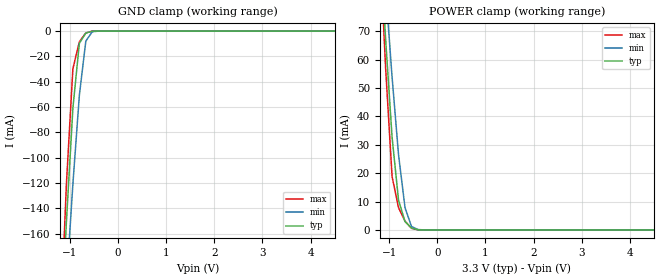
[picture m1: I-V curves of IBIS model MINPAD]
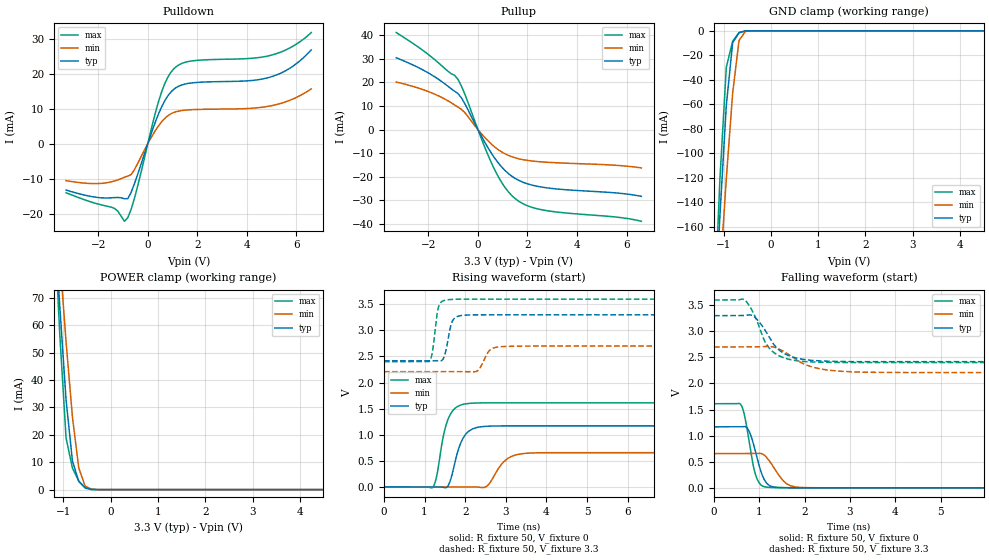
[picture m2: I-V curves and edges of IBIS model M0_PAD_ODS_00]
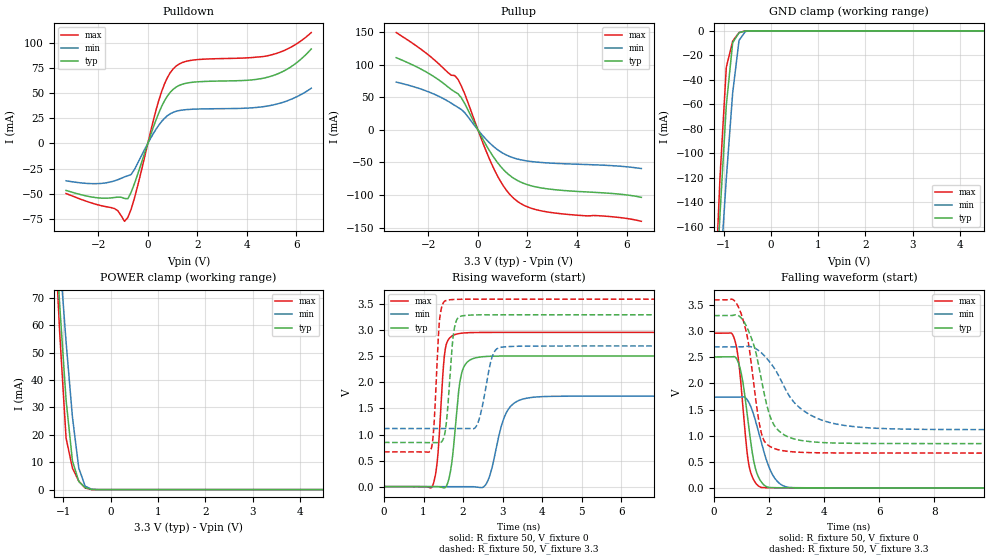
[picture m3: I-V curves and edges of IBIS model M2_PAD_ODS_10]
| Created by SiliconSmart  O-2018.09-SP2-3
[IBIS Ver]   4.0
[File Name]   as31b32bc_3p3_rev1p4.ibs
[File Rev]   1.4
[Date]   Thursday Mar 21 2024
|[Source]   Avalanche Team
|[Notes]   Generated IBIS models from Silicon Smart
|[Rev 1.0]  Initial Release based on extracted netlist
|   Characterization
|[Rev 1.1]  Recharacterization with Hspice, run in high accuracy mode
|[Rev 1.2]  Recharacterization with Hspice, run with parameters inline
|   with the datasheet
|[Rev 1.3]  Recharacterization with Hspice, run with updated VIH/VIL
|   in parallel with datasheet rev X.7
|[Rev 1.4]  Update the pin to the package pinout assignment
|[Disclaimer]   THE MODEL LIBRARIES ARE PROVIDED AS IS.
|[Copyright]   Copyright 2019, Avalanche Technology., All Rights Reserved
[Component]   AS301GB32_BGA
[Manufacturer] Avalanche Technology
| CONTENT :
| This file contains IBIS MODEL for PSRAM device
| AS301GB32
| USAGE :
| The models are derived for the 2.7V to 3.6V I/O Operation.
| Temperatures for model generation: typ: 25, max: -40, min: 125
| Voltages : typ: 3.3V, min: 2.7V, max: 3.6V
| PACKAGES SUPPORTED :
| 142-ball FBGA (15mm x 17mm)
| VERIFICATION
| Errors  : 0
| Warnings: 11
| All warnings due to non-monotonic data:
[Package]
R_pkg  0   0   0
L_pkg  0   0   0
C_pkg  0   0   0
[Pin]   signal_name   model_name   R_pin   L_pin   C_pin
P8   E#   MINPAD   0.254	7.307E-9	1.178E-12
P7   G#   MINPAD   0.243	7.052E-9	1.094E-12
J2   CR#   MINPAD   0.547	10.386E-9	1.789E-12
K3   PG#   MINPAD   0.451	10.329E-9	1.676E-12
M8   W#   MINPAD   0.377	9.020E-9	1.417E-12
M2   ADDR_26   MINPAD   0.425	9.037E-9	1.604E-12
L4   ADDR_25   MINPAD   0.419	9.644E-9	1.527E-12
K13   ADDR_24   MINPAD   0.495	9.978E-9	1.745E-12
M3   ADDR_23   MINPAD   0.371	9.313E-9	1.466E-12
L3   ADDR_22   MINPAD   0.412	9.753E-9	1.540E-12
M7   ADDR_21   MINPAD   0.368	8.765E-9	1.384E-12
P12   ADDR_20   MINPAD   0.287	8.287E-9	1.639E-12
L12   ADDR_19   MINPAD   0.424	10.320E-9	1.620E-12
N11   ADDR_18   MINPAD   0.338	8.691E-9	1.470E-12
N6   ADDR_17   MINPAD   0.309	8.196E-9	1.279E-12
P6   ADDR_16   MINPAD   0.256	7.462E-9	1.204E-12
L13   ADDR_15   MINPAD   0.463	10.719E-9	1.740E-12
M13   ADDR_14   MINPAD   0.421	10.290E-9	1.689E-12
P10   ADDR_13   MINPAD   0.262	7.671E-9	1.349E-12
N10   ADDR_12   MINPAD   0.340	8.540E-9	1.360E-12
M12   ADDR_11   MINPAD   0.402	9.876E-9	1.604E-12
N13   ADDR_10   MINPAD   0.399	9.819E-9	1.696E-12
L11   ADDR_9   MINPAD   0.443	9.732E-9	1.569E-12
M11   ADDR_8   MINPAD   0.436	9.682E-9	1.671E-12
P5   ADDR_7   MINPAD   0.253	7.464E-9	1.277E-12
P3   ADDR_6   MINPAD   0.279	8.031E-9	1.557E-12
N5   ADDR_5   MINPAD   0.313	8.320E-9	1.359E-12
N4   ADDR_4   MINPAD   0.329	8.138E-9	1.428E-12
M4   ADDR_3   MINPAD   0.379	8.543E-9	1.406E-12
N2   ADDR_2   MINPAD   0.378	9.572E-9	1.637E-12
N9   ADDR_1   MINPAD   0.315	8.416E-9	1.305E-12
M9   ADDR_0   MINPAD   0.403	9.225E-9	1.473E-12
E2   DQ_31   MIOPAD   0.365	8.798E-9	1.454E-12
F2   DQ_30   MIOPAD   0.418	9.057E-9	1.576E-12
D2   DQ_29   MIOPAD   0.358	8.697E-9	1.520E-12
E3   DQ_28   MIOPAD   0.348	8.812E-9	1.441E-12
E12   DQ_27   MIOPAD   0.327	8.506E-9	1.443E-12
D10   DQ_26   MIOPAD   0.309	7.715E-9	1.264E-12
C9   DQ_25   MIOPAD   0.279	7.395E-9	1.219E-12
C7   DQ_24   MIOPAD   0.252	6.802E-9	1.108E-12
G4   DQ_23   MIOPAD   0.455	10.071E-9	1.775E-12
G3   DQ_22   MIOPAD   0.457	10.100E-9	1.750E-12
F13   DQ_21   MIOPAD   0.377	9.387E-9	1.566E-12
D13   DQ_20   MIOPAD   0.295	8.231E-9	1.460E-12
C10   DQ_19   MIOPAD   0.293	7.553E-9	1.298E-12
E8   DQ_18   MIOPAD   0.393	8.323E-9	1.436E-12
F6   DQ_17   MIOPAD   0.425	8.913E-9	1.517E-12
E5   DQ_16   MIOPAD   0.379	8.982E-9	1.460E-12
E13   DQ_15   MIOPAD   0.363	8.555E-9	1.474E-12
G11   DQ_14   MIOPAD   0.475	9.536E-9	1.630E-12
E10   DQ_13   MIOPAD   0.404	8.563E-9	1.453E-12
F9   DQ_12   MIOPAD   0.409	9.347E-9	1.513E-12
C8   DQ_11   MIOPAD   0.257	6.782E-9	1.111E-12
C6   DQ_10   MIOPAD   0.238	7.000E-9	1.114E-12
D6   DQ_9   MIOPAD   0.292	7.776E-9	1.248E-12
D4   DQ_8   MIOPAD   0.305	7.782E-9	1.343E-12
G12   DQ_7   MIOPAD   0.502	10.055E-9	1.687E-12
C12   DQ_6   MIOPAD   0.275	7.857E-9	1.346E-12
D11   DQ_5   MIOPAD   0.286	7.835E-9	1.360E-12
D9   DQ_4   MIOPAD   0.306	8.035E-9	1.299E-12
E7   DQ_3   MIOPAD   0.384	8.178E-9	1.375E-12
C5   DQ_2   MIOPAD   0.231	6.786E-9	1.150E-12
D5   DQ_1   MIOPAD   0.307	7.698E-9	1.346E-12
C3   DQ_0   MIOPAD   0.267	7.420E-9	1.241E-12
G13   INT#   MIOPAD   0.480	10.704E-9	1.759E-12
F10   VSSIO   GND   NA   NA   NA
L10   VSSIO   GND   NA   NA   NA
E9   VSSIO   GND   NA   NA   NA
L9   VSSIO   GND   NA   NA   NA
F8   VSSIO   GND   NA   NA   NA
L8   VSSIO   GND   NA   NA   NA
F7   VSSIO   GND   NA   NA   NA
L7   VSSIO   GND   NA   NA   NA
E6   VSSIO   GND   NA   NA   NA
L6   VSSIO   GND   NA   NA   NA
G5   VSSIO   GND   NA   NA   NA
A14   VSS   GND   NA   NA   NA
B14   VSS   GND   NA   NA   NA
C14   VSS   GND   NA   NA   NA
H13   VSS   GND   NA   NA   NA
R14   VSS   GND   NA   NA   NA
T14   VSS   GND   NA   NA   NA
A13   VSS   GND   NA   NA   NA
T13   VSS   GND   NA   NA   NA
A12   VSS   GND   NA   NA   NA
G10   VSS   GND   NA   NA   NA
H10   VSS   GND   NA   NA   NA
J10   VSS   GND   NA   NA   NA
K10   VSS   GND   NA   NA   NA
F5   VSS   GND   NA   NA   NA
L5   VSS   GND   NA   NA   NA
A2   VSS   GND   NA   NA   NA
T2   VSS   GND   NA   NA   NA
A1   VSS   GND   NA   NA   NA
B1   VSS   GND   NA   NA   NA
R1   VSS   GND   NA   NA   NA
T1   VSS   GND   NA   NA   NA
F12   VCCIO   POWER   NA   NA   NA
J12   VCCIO   POWER   NA   NA   NA
E11   VCCIO   POWER   NA   NA   NA
M10   VCCIO   POWER   NA   NA   NA
D8   VCCIO   POWER   NA   NA   NA
N8   VCCIO   POWER   NA   NA   NA
D7   VCCIO   POWER   NA   NA   NA
N7   VCCIO   POWER   NA   NA   NA
M5   VCCIO   POWER   NA   NA   NA
E4   VCCIO   POWER   NA   NA   NA
F3   VCCIO   POWER   NA   NA   NA
J3   VCCIO   POWER   NA   NA   NA
C13   VCC   POWER   NA   NA   NA
P13   VCC   POWER   NA   NA   NA
D12   VCC   POWER   NA   NA   NA
N12   VCC   POWER   NA   NA   NA
C11   VCC   POWER   NA   NA   NA
F11   VCC   POWER   NA   NA   NA
H11   VCC   POWER   NA   NA   NA
J11   VCC   POWER   NA   NA   NA
K11   VCC   POWER   NA   NA   NA
P11   VCC   POWER   NA   NA   NA
C4   VCC   POWER   NA   NA   NA
F4   VCC   POWER   NA   NA   NA
H4   VCC   POWER   NA   NA   NA
J4   VCC   POWER   NA   NA   NA
K4   VCC   POWER   NA   NA   NA
P4   VCC   POWER   NA   NA   NA
D3   VCC   POWER   NA   NA   NA
N3   VCC   POWER   NA   NA   NA
C2   VCC   POWER   NA   NA   NA
P2   VCC   POWER   NA   NA   NA
| IOPAD
[Model Selector] MIOPAD
| Model Description
M0_PAD_ODS_00   ODS_00
M1_PAD_ODS_01   ODS_01
M2_PAD_ODS_10   ODS_10
M3_PAD_ODS_11   ODS_11
| Models and submodels in the file (5): MINPAD (Input), M0_PAD_ODS_00 (I/O), M2_PAD_ODS_10 (I/O), M1_PAD_ODS_01 (I/O), M3_PAD_ODS_11 (I/O)
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[Model] MINPAD
Model_type Input
Enable   Active-High
Vinl  =  0.8
Vinh  =  2.2
| Capacitance  typ   min   max
C_comp   1.514821e-12   1.418868e-12   1.647023e-12
| Variables   typ   min   max
[GND Clamp Reference]   0   0   0
[POWER Clamp Reference]   3.3   2.7   3.6
[Pulldown Reference]   0   0   0
[Pullup Reference]   3.3   2.7   3.6
[Temperature Range]   25   125   -40
[Voltage Range]   3.3   2.7   3.6
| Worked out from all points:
|   GND clamp passes 1 mA (typ) near -0.62 V on its own axis
|   POWER clamp passes 1 mA (typ) near -0.56 V on its own axis
[GND Clamp]
| Voltage   I(typ)   I(min)   I(max)
-3.3V     -1.961A    -1.697A    -2.357A
-1.21V    -250.7mA   -283.7mA   -242.5mA
-1.076V   -150.6mA   -200.1mA   -120.6mA
-941.4mV  -60.83mA   -120.8mA   -29.75mA
-806.9mV  -9.646mA   -50.71mA   -8.435mA
-672.4mV  -1.585mA   -7.866mA   -1.457mA
-537.9mV  -71.75uA   -504.3uA   -18.73uA
-403.4mV  -593.9nA   -18.57uA   -37.22nA
6.6V      0A         0A         0A
[POWER Clamp]
| Voltage   I(typ)   I(min)   I(max)
-3.3V     772.3mA    673.3mA    930.5mA
-1.21V    105.9mA    117.6mA    104.6mA
-1.076V   67.34mA    85.06mA    57.16mA
-941.4mV  32.71mA    53.93mA    18.82mA
-806.9mV  10.48mA    26.53mA    7.848mA
-672.4mV  2.975mA    7.856mA    3.108mA
-537.9mV  710.9uA    1.248mA    573.1uA
-403.4mV  60.69uA    160.8uA    9.187uA
-269mV    142.4nA    6.118uA    23.26nA
6.6V      0A         0A         0A
[Model] M0_PAD_ODS_00
Model_type I/O
Enable   Active-High
Vinl  =  0.8
Vinh  =  2.2
Vmeas =  1.65
Cref  =  30e-12
| Capacitance  typ   min   max
C_comp   1.518749e-12   1.424706e-12   1.652746e-12
| Variables   typ   min   max
[GND Clamp Reference]   0   0   0
[POWER Clamp Reference]   3.3   2.7   3.6
[Pulldown Reference]   0   0   0
[Pullup Reference]   3.3   2.7   3.6
[Temperature Range]   25   125   -40
[Voltage Range]   3.3   2.7   3.6
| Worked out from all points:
|   slope of the pulldown table from 0 to 0.495 V, typ, clamps not added: 52.1 ohm
|   slope of the pullup table from 0 to 0.495 V, typ, clamps not added: 53.8 ohm
|   GND clamp passes 1 mA (typ) near -0.62 V on its own axis
|   POWER clamp passes 1 mA (typ) near -0.56 V on its own axis
|   falling waveform, R_fixture 50, V_fixture 0: 20-80 % time 230ps typ, 320ps min, 198ps max; typ from 1.17 V to 0 V
|   falling waveform, R_fixture 50, V_fixture 3.3: 20-80 % time 464ps typ, 644ps min, 396ps max; typ from 3.3 V to 2.42 V
|   rising waveform, R_fixture 50, V_fixture 0: 20-80 % time 273ps typ, 362ps min, 248ps max; typ from 0 V to 1.17 V
|   rising waveform, R_fixture 50, V_fixture 3.3: 20-80 % time 138ps typ, 198ps min, 114ps max; typ from 2.42 V to 3.3 V
[GND Clamp]
| Voltage   I(typ)   I(min)   I(max)
-3.3V     -1.961A    -1.697A    -2.357A
-1.21V    -250.7mA   -283.7mA   -242.5mA
-1.076V   -150.6mA   -200.1mA   -120.7mA
-941.4mV  -60.83mA   -120.8mA   -29.76mA
-806.9mV  -9.649mA   -50.71mA   -8.442mA
-672.4mV  -1.587mA   -7.866mA   -1.46mA
-537.9mV  -71.93uA   -504.3uA   -18.83uA
-403.4mV  -595.6nA   -18.58uA   -37.45nA
6.6V      0A         0A         0A
[POWER Clamp]
| Voltage   I(typ)   I(min)   I(max)
-3.3V     772.3mA    673.3mA    930.5mA
-1.21V    105.9mA    117.6mA    104.6mA
-1.076V   67.34mA    85.06mA    57.16mA
-941.4mV  32.71mA    53.93mA    18.82mA
-806.9mV  10.48mA    26.53mA    7.848mA
-672.4mV  2.975mA    7.856mA    3.108mA
-537.9mV  710.9uA    1.248mA    573.1uA
-403.4mV  60.69uA    160.8uA    9.187uA
-269mV    142.4nA    6.118uA    23.26nA
6.6V      0A         0A         0A
[Pulldown]
| Voltage   I(typ)   I(min)   I(max)
-3.3V     -13.26mA   -10.58mA   -14.05mA
-1.345V   -15.42mA   -10.67mA   -18.51mA
-941.4mV  -15.74mA   -9.611mA   -22.19mA
-806.9mV  -15.73mA   -9.263mA   -21.14mA
-537.9mV  -11.42mA   -7.417mA   -15.59mA
455.2mV   8.881mA    5.308mA    12.55mA
682.8mV   12.23mA    7.205mA    17.1mA
1.024V    15.38mA    8.837mA    21.2mA
1.821V    17.39mA    9.724mA    23.68mA
4.914V    18.96mA    10.73mA    25.16mA
5.783V    21.77mA    12.53mA    27.53mA
6.6V      26.8mA     15.66mA    31.75mA
[Pullup]
| Voltage   I(typ)   I(min)   I(max)
-3.3V     30.44mA    20.14mA    41.1mA
-1.883V   23.26mA    15.61mA    30.81mA
-806.9mV  15.23mA    9.539mA    21.27mA
-537.9mV  11.14mA    7.294mA    15.26mA
227.6mV   -4.448mA   -2.796mA   -6.209mA
682.8mV   -12.17mA   -7.42mA    -17.15mA
1.138V    -17.78mA   -10.49mA   -25.16mA
1.593V    -21.21mA   -12.21mA   -29.96mA
2.048V    -23.14mA   -13.13mA   -32.47mA
2.731V    -24.61mA   -13.8mA    -34.27mA
5.659V    -26.92mA   -15.2mA    -37.16mA
6.6V      -28.29mA   -16.23mA   -38.86mA
[Ramp]
dV/dt_r   0.701574/0.273396n  0.393696/0.362182n  0.967082/0.24767n
dV/dt_f   0.529393/0.463707n  0.294233/0.644316n  0.719379/0.396117n
R_load = 50
[Falling Waveform]
R_fixture = 50
V_fixture = 0
V_fixture_min = 0
V_fixture_max = 0
| Time   V(typ)   V(min)   V(max)
0s        1.169V     656.2mV    1.612V
592.6ps   1.17V      656.6mV    1.594V
662.7ps   1.175V     656.6mV    1.423V
757.8ps   1.11V      656.7mV    979.6mV
920.8ps   673.8mV    658.3mV    236.4mV
1.068ns   233.8mV    649.1mV    35.66mV
1.221ns   45.34mV    516.2mV    8.708mV
1.592ns   3.21mV     87.01mV    1.102mV
2.018ns   581.9uV    4.7mV      706uV
21.88ns   211nV      -2.279uV   3.818uV
[Falling Waveform]
R_fixture = 50
V_fixture = 3.3
V_fixture_min = 2.7
V_fixture_max = 3.6
| Time   V(typ)   V(min)   V(max)
0s        3.3V       2.7V       3.6V
662.6ps   3.302V     2.701V     3.609V
894.9ps   3.273V     2.701V     3.302V
1.117ns   3.036V     2.709V     2.815V
1.233ns   2.866V     2.709V     2.664V
1.51ns    2.594V     2.628V     2.502V
2.006ns   2.457V     2.366V     2.42V
2.5ns     2.427V     2.259V     2.405V
3.502ns   2.418V     2.214V     2.401V
21.88ns   2.418V     2.21V      2.401V
[Rising Waveform]
R_fixture = 50
V_fixture = 0
V_fixture_min = 0
V_fixture_max = 0
| Time   V(typ)   V(min)   V(max)
0s        11.89nV    88.47nV    -73.19nV
1.207ns   -862.4uV   -520.5uV   -4.427mV
1.285ns   -918.3uV   -554.2uV   157.9mV
1.593ns   39.36mV    -686.9uV   1.324V
1.858ns   773.7mV    -801.1uV   1.558V
2.069ns   1.055V     -892.4uV   1.599V
2.519ns   1.162V     5.17mV     1.611V
2.991ns   1.169V     510.2mV    1.611V
3.605ns   1.169V     648.6mV    1.611V
21.88ns   1.169V     656.2mV    1.612V
[Rising Waveform]
R_fixture = 50
V_fixture = 3.3
V_fixture_min = 2.7
V_fixture_max = 3.6
| Time   V(typ)   V(min)   V(max)
0s        2.418V     2.21V      2.401V
1.115ns   2.419V     2.21V      2.406V
1.19ns    2.419V     2.21V      2.571V
1.354ns   2.418V     2.21V      3.473V
1.494ns   2.522V     2.21V      3.578V
1.647ns   3.091V     2.21V      3.594V
2.284ns   3.299V     2.216V     3.599V
2.637ns   3.299V     2.641V     3.599V
3.102ns   3.299V     2.696V     3.599V
21.88ns   3.3V       2.7V       3.6V
[Model] M2_PAD_ODS_10
Model_type I/O
Enable   Active-High
Vinl  =  0.8
Vinh  =  2.2
Vmeas =  1.65
Cref  =  30e-12
| Capacitance  typ   min   max
C_comp   1.518749e-12   1.424706e-12   1.652746e-12
| Variables   typ   min   max
[GND Clamp Reference]   0   0   0
[POWER Clamp Reference]   3.3   2.7   3.6
[Pulldown Reference]   0   0   0
[Pullup Reference]   3.3   2.7   3.6
[Temperature Range]   25   125   -40
[Voltage Range]   3.3   2.7   3.6
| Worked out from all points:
|   slope of the pulldown table from 0 to 0.495 V, typ, clamps not added: 14.9 ohm
|   slope of the pullup table from 0 to 0.495 V, typ, clamps not added: 14.7 ohm
|   GND clamp passes 1 mA (typ) near -0.62 V on its own axis
|   POWER clamp passes 1 mA (typ) near -0.56 V on its own axis
|   falling waveform, R_fixture 50, V_fixture 0: 20-80 % time 394ps typ, 590ps min, 315ps max; typ from 2.51 V to 0 V
|   falling waveform, R_fixture 50, V_fixture 3.3: 20-80 % time 660ps typ, 1.32ns min, 479ps max; typ from 3.3 V to 0.848 V
|   rising waveform, R_fixture 50, V_fixture 0: 20-80 % time 197ps typ, 348ps min, 149ps max; typ from 0 V to 2.51 V
|   rising waveform, R_fixture 50, V_fixture 3.3: 20-80 % time 147ps typ, 240ps min, 115ps max; typ from 0.848 V to 3.3 V
[GND Clamp]
| Voltage   I(typ)   I(min)   I(max)
-3.3V     -1.961A    -1.697A    -2.357A
-1.21V    -250.7mA   -283.7mA   -242.5mA
-1.076V   -150.6mA   -200.1mA   -120.7mA
-941.4mV  -60.83mA   -120.8mA   -29.76mA
-806.9mV  -9.649mA   -50.71mA   -8.442mA
-672.4mV  -1.587mA   -7.866mA   -1.46mA
-537.9mV  -71.93uA   -504.3uA   -18.83uA
-403.4mV  -595.6nA   -18.58uA   -37.45nA
6.6V      0A         0A         0A
[POWER Clamp]
| Voltage   I(typ)   I(min)   I(max)
-3.3V     772.3mA    673.3mA    930.5mA
-1.21V    105.9mA    117.6mA    104.6mA
-1.076V   67.34mA    85.06mA    57.16mA
-941.4mV  32.71mA    53.93mA    18.82mA
-806.9mV  10.48mA    26.53mA    7.848mA
-672.4mV  2.975mA    7.856mA    3.108mA
-537.9mV  710.9uA    1.248mA    573.1uA
-403.4mV  60.69uA    160.8uA    9.187uA
-269mV    142.4nA    6.118uA    23.26nA
6.6V      0A         0A         0A
[Pulldown]
| Voltage   I(typ)   I(min)   I(max)
-3.3V     -46.77mA   -37.16mA   -49.83mA
-1.345V   -53.76mA   -37.21mA   -64.77mA
-941.4mV  -54.71mA   -33.33mA   -77.43mA
-806.9mV  -55.02mA   -32.17mA   -73.73mA
-537.9mV  -39.9mA    -25.92mA   -54.28mA
455.2mV   31.02mA    18.55mA    43.7mA
682.8mV   42.73mA    25.18mA    59.65mA
1.024V    53.77mA    30.89mA    74.07mA
1.821V    60.81mA    33.99mA    82.81mA
4.914V    66.31mA    37.51mA    87.55mA
5.783V    76.16mA    43.8mA     95.68mA
6.6V      93.82mA    54.81mA    110.2mA
[Pullup]
| Voltage   I(typ)   I(min)   I(max)
-3.3V     110.8mA    73.4mA     149.4mA
-1.883V   84.27mA    56.72mA    111.4mA
-806.9mV  55.48mA    34.56mA    77.7mA
-537.9mV  40.72mA    26.67mA    55.72mA
227.6mV   -16.26mA   -10.22mA   -22.67mA
682.8mV   -44.48mA   -27.12mA   -62.65mA
1.138V    -65.01mA   -38.35mA   -91.97mA
1.593V    -77.56mA   -44.65mA   -109.6mA
2.162V    -85.85mA   -48.54mA   -120.3mA
2.845V    -90.61mA   -50.73mA   -126.1mA
5.534V    -97.91mA   -55.15mA   -133.7mA
6.6V      -103.4mA   -59.29mA   -140.2mA
[Ramp]
dV/dt_r   1.50494/0.197293n  1.04234/0.347547n  1.77705/0.14905n
dV/dt_f   1.47118/0.66022n  0.951015/1.316n  1.76015/0.479444n
R_load = 50
[Falling Waveform]
R_fixture = 50
V_fixture = 0
V_fixture_min = 0
V_fixture_max = 0
| Time   V(typ)   V(min)   V(max)
0s        2.508V     1.737V     2.962V
759.6ps   2.508V     1.738V     2.821V
890.4ps   2.387V     1.738V     2.436V
999.8ps   2.164V     1.741V     1.857V
1.254ns   1.197V     1.646V     471.7mV
1.462ns   460.6mV    1.364V     132.2mV
1.72ns    111.8mV    859.7mV    7.736mV
2.149ns   3.807mV    230.1mV    1.501mV
2.718ns   1.059mV    9.353mV    845.9uV
21.88ns   537.2nV    325.5nV    -804nV
[Falling Waveform]
R_fixture = 50
V_fixture = 3.3
V_fixture_min = 2.7
V_fixture_max = 3.6
| Time   V(typ)   V(min)   V(max)
0s        3.3V       2.7V       3.6V
659.1ps   3.3V       2.7V       3.614V
907.4ps   3.292V     2.701V     3.438V
1.244ns   3.017V     2.711V     2.79V
1.71ns    2.099V     2.591V     1.067V
2ns       1.425V     2.426V     802.7mV
2.308ns   1.117V     2.186V     732.6mV
3.226ns   902.4mV    1.487V     679.2mV
4.9ns     853.7mV    1.183V     667.3mV
21.88ns   848mV      1.115V     666.4mV
[Rising Waveform]
R_fixture = 50
V_fixture = 0
V_fixture_min = 0
V_fixture_max = 0
| Time   V(typ)   V(min)   V(max)
0s        5.777nV    44.9nV     -42.68nV
1.217ns   886.5uV    -289.8uV   -4.263mV
1.357ns   1.052mV    -323.2uV   556.4mV
1.551ns   -16.19mV   -369.6uV   2.647V
1.711ns   437.6mV    -407.7uV   2.887V
1.916ns   1.993V     -456.6uV   2.942V
2.553ns   2.498V     17.69mV    2.961V
3.099ns   2.508V     1.428V     2.962V
3.73ns    2.508V     1.712V     2.962V
21.88ns   2.508V     1.737V     2.962V
[Rising Waveform]
R_fixture = 50
V_fixture = 3.3
V_fixture_min = 2.7
V_fixture_max = 3.6
| Time   V(typ)   V(min)   V(max)
0s        848mV      1.115V     666.4mV
1.189ns   847.3mV    1.116V     714.5mV
1.41ns    844.8mV    1.116V     3.235V
1.604ns   1.442V     1.116V     3.581V
1.773ns   3.011V     1.116V     3.594V
2.021ns   3.283V     1.116V     3.599V
2.351ns   3.297V     1.183V     3.599V
2.742ns   3.299V     2.508V     3.599V
3.026ns   3.299V     2.682V     3.599V
21.88ns   3.3V       2.7V       3.6V
